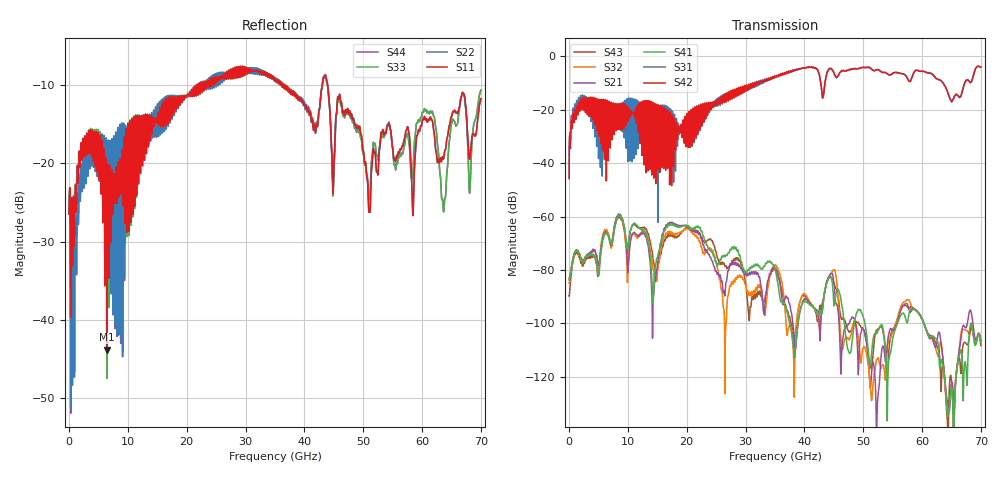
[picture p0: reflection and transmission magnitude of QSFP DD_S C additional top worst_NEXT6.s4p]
! AWR Design Environment (8415) Fri Dec 21 09:11:22 2018
! Document = 'CHANNEL TEST'
! nPorts: 4, nXvals: 7001
# HZ S DB R 50
!Freq DBS11 AngS11 DBS12 AngS12 DBS13 AngS13 DBS14 AngS14
!	DBS21 AngS21 DBS22 AngS22 DBS23 AngS23 DBS24 AngS24
!	DBS31 AngS31 DBS32 AngS32 DBS33 AngS33 DBS34 AngS34
!	DBS41 AngS41 DBS42 AngS42 DBS43 AngS43 DBS44 AngS44
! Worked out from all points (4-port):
!   7000 points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, 10 MHz to 70 GHz, reference 50 ohm
!   strongest paths, dB at 10 MHz, 17.51 GHz, 35.01 GHz, 52.51 GHz, 70 GHz:
!     S42: -45.8, -24.5, -7.4, -5.0, -4.0
!     S31: -45.1, -23.1, -7.6, -5.0, -4.0
!     S41: -83.8, -62.5, -79.6, -102.8, -107.2
!     S21: -83.1, -62.2, -79.2, -127.1, -106.3
!     S32: -84.9, -66.0, -78.3, -112.9, -107.4
!     S43: -89.7, -66.7, -80.0, -102.0, -108.3
!   lowest |S11| = -43.8 dB at 6.41 GHz (marker M1), VSWR 1.01, Z = 50.5 - j0.428 ohm
!   |S11| at or under -10 dB: start of sweep to 21.78 GHz; 36.52 GHz to 43.04 GHz (6.515 GHz wide, 16.4 % of centre); 43.91 GHz to end of sweep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
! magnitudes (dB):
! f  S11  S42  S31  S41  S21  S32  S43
! 10 MHz  -26.5  -45.8  -45.1  -83.8  -83.1  -84.9  -89.7
! 1.65 GHz  -19.9  -17.1  -15.4  -73.7  -73.6  -74.1  -75.0
! 6.41 GHz  -43.8  -20.4  -18.7  -66.2  -66.0  -65.0  -65.3
! 18.4 GHz  -11.6  -29.7  -32.9  -63.8  -63.2  -66.4  -67.5
! 30.78 GHz  -8.1  -11.1  -11.9  -79.3  -81.2  -88.6  -93.7
! 63.65 GHz  -19.4  -10.2  -10.2  -116.7  -115.2  -116.8  -116.4
! 70 GHz  -11.8  -4.0  -4.0  -107.2  -106.3  -107.4  -108.3
